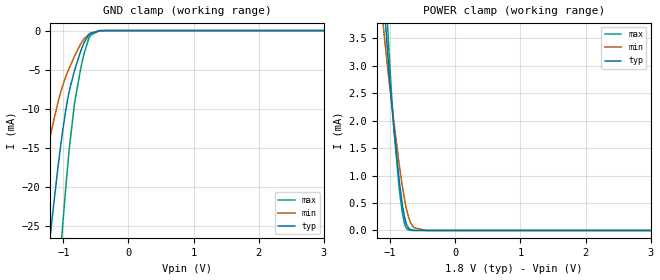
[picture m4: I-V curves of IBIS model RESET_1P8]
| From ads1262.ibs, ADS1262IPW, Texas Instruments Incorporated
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|   Model RESET_1P8
[Model]   RESET_1P8
Model_type   Input
Vinl = 0.36
Vinh = 1.44
|   typ   min   max
|   (nom PVT)   (fast PVT)   (slow PVT)
C_comp   0.205pF   0.203pF   0.216pF
[Model spec]
|subparameter
Vinl   0.36   0.33   0.39
Vinh   1.44   1.32   1.56
[Voltage Range]   1.8   1.65   1.95
[Temperature Range]   27   125   -40
[Power Clamp Reference]   1.8   1.65   1.95
[GND Clamp Reference]   -0   -0   -0
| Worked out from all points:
|   GND clamp passes 1 mA (typ) near -0.64 V on its own axis
|   POWER clamp passes 1 mA (typ) near -0.87 V on its own axis
[GND Clamp]
|   Voltage   I(typ)   I(min)   I(max)
-1.8V     -82.47mA   -44.96mA   -122.6mA
-1.552V   -57.7mA    -30.44mA   -90.58mA
-1.417V   -44.97mA   -23.36mA   -73.38mA
-1.217V   -27.66mA   -14.22mA   -48.58mA
-1.168V   -23.83mA   -12.29mA   -42.77mA
-1.017V   -13.3mA    -7.247mA   -25.72mA
-903.6mV  -7.563mA   -4.715mA   -14.77mA
-828mV    -5.119mA   -3.297mA   -9.329mA
-687.6mV  -1.673mA   -1.122mA   -3.161mA
-585mV    -343uA     -366.7uA   -623.2uA
-417.6mV  -5.153uA   -30.77uA   -4.357uA
3.595V    0A         0A         0A
[POWER Clamp]
|   Voltage   I(typ)   I(min)   I(max)
-1.8V     18.43mA    14.33mA    22.64mA
-1.157V   5.308mA    4.346mA    6.439mA
-1.082V   3.943mA    3.437mA    4.663mA
-1.044V   3.313mA    3.017mA    3.817mA
-1.022V   2.974mA    2.785mA    3.352mA
-941.4mV  1.845mA    1.955mA    1.823mA
-860.4mV  906uA      1.197mA    758.9uA
-806.4mV  420.7uA    756.1uA    277.6uA
-736.2mV  77.89uA    320.8uA    22.95uA
-639mV    2.656uA    53.3uA     325.4nA
-450mV    0A         339.1nA    0A
3.595V    0A         0A         0A
